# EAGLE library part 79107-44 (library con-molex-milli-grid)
RECEPTACAL
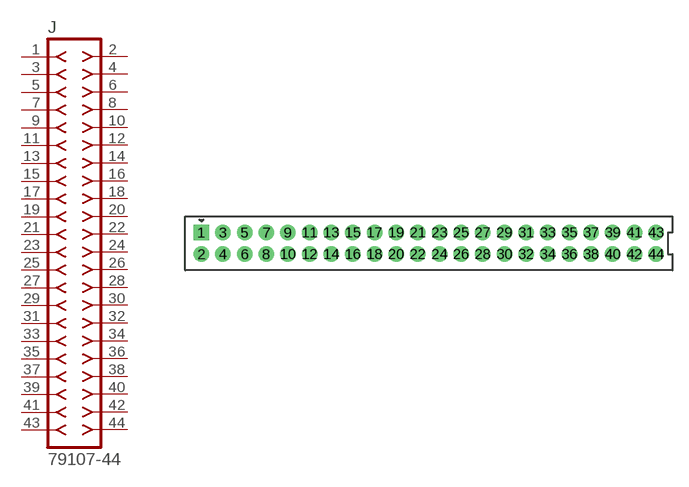
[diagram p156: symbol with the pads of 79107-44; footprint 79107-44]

Designator prefix J

## 79107-44  [79107-44]
1  1  pas
2  2  pas
3  3  pas
4  4  pas
5  5  pas
6  6  pas
7  7  pas
8  8  pas
9  9  pas
10  10  pas
11  11  pas
12  12  pas
13  13  pas
14  14  pas
15  15  pas
16  16  pas
17  17  pas
18  18  pas
19  19  pas
20  20  pas
21  21  pas
22  22  pas
23  23  pas
24  24  pas
25  25  pas
26  26  pas
27  27  pas
28  28  pas
29  29  pas
30  30  pas
31  31  pas
32  32  pas
33  33  pas
34  34  pas
35  35  pas
36  36  pas
37  37  pas
38  38  pas
39  39  pas
40  40  pas
41  41  pas
42  42  pas
43  43  pas
44  44  pas

## Footprint 79107-44 (pad centres in mm)
RECEPTACAL Dual Row, Vertical, Through-Hole
drill 0.914 square: 1 -21,1
drill 0.914: 2 -21,-1; 3 -19,1; 4 -19,-1; 5 -17,1; 6 -17,-1; 7 -15,1; 8 -15,-1; 9 -13,1; 10 -13,-1; 11 -11,1; 12 -11,-1; 13 -9,1; 14 -9,-1; 15 -7,1; 16 -7,-1; 17 -5,1; 18 -5,-1; 19 -3,1; 20 -3,-1; 21 -1,1; 22 -1,-1; 23 1,1; 24 1,-1; 25 3,1; 26 3,-1; 27 5,1; 28 5,-1; 29 7,1; 30 7,-1; 31 9,1; 32 9,-1; 33 11,1; 34 11,-1; 35 13,1; 36 13,-1; 37 15,1; 38 15,-1; 39 17,1; 40 17,-1; 41 19,1; 42 19,-1; 43 21,1; 44 21,-1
